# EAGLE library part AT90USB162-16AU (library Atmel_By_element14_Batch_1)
8-bit Microcontroller
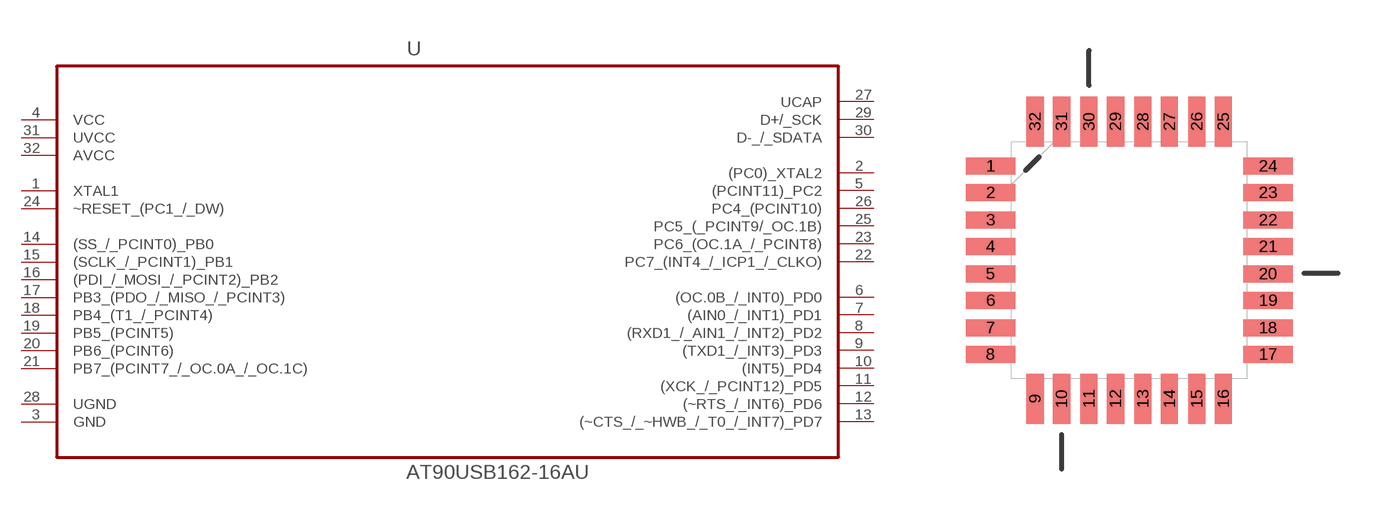
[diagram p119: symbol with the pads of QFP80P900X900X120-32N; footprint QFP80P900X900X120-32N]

Designator prefix U

## AT90USB162-16AU (MPN: AT90USB162-16AU; OC_FARNELL: 1455073; OC_NEWARK: 58M3868; PACKAGE: TQFP-32; SUPPLIER: Atmel)  [QFP80P900X900X120-32N]
1  XTAL1  in
2  (PC0)_XTAL2
3  GND  pas
4  VCC  pwr
5  (PCINT11)_PC2
6  (OC.0B_/_INT0)_PD0
7  (AIN0_/_INT1)_PD1
8  (RXD1_/_AIN1_/_INT2)_PD2
9  (TXD1_/_INT3)_PD3
10  (INT5)_PD4
11  (XCK_/_PCINT12)_PD5
12  (~RTS_/_INT6)_PD6
13  (~CTS_/_~HWB_/_T0_/_INT7)_PD7
14  (SS_/_PCINT0)_PB0
15  (SCLK_/_PCINT1)_PB1
16  (PDI_/_MOSI_/_PCINT2)_PB2
17  PB3_(PDO_/_MISO_/_PCINT3)
18  PB4_(T1_/_PCINT4)
19  PB5_(PCINT5)
20  PB6_(PCINT6)
21  PB7_(PCINT7_/_OC.0A_/_OC.1C)
22  PC7_(INT4_/_ICP1_/_CLKO)
23  PC6_(OC.1A_/_PCINT8)
24  ~RESET_(PC1_/_DW)
25  PC5_(_PCINT9/_OC.1B)
26  PC4_(PCINT10)
27  UCAP  out
28  UGND  pas
29  D+/_SCK
30  D-_/_SDATA
31  UVCC  pwr
32  AVCC  pwr

## Footprint QFP80P900X900X120-32N (pad centres in mm)
smd 1.473 x 0.508: 1 -4.115,2.794; 2 -4.115,2.007; 3 -4.115,1.194; 4 -4.115,0.406; 5 -4.115,-0.406; 6 -4.115,-1.194; 7 -4.115,-2.007; 8 -4.115,-2.794; 17 4.115,-2.794; 18 4.115,-2.007; 19 4.115,-1.194; 20 4.115,-0.406; 21 4.115,0.406; 22 4.115,1.194; 23 4.115,2.007; 24 4.115,2.794
smd 0.508 x 1.473: 9 -2.794,-4.115; 10 -2.007,-4.115; 11 -1.194,-4.115; 12 -0.406,-4.115; 13 0.406,-4.115; 14 1.194,-4.115; 15 2.007,-4.115; 16 2.794,-4.115; 25 2.794,4.115; 26 2.007,4.115; 27 1.194,4.115; 28 0.406,4.115; 29 -0.406,4.115; 30 -1.194,4.115; 31 -2.007,4.115; 32 -2.794,4.115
